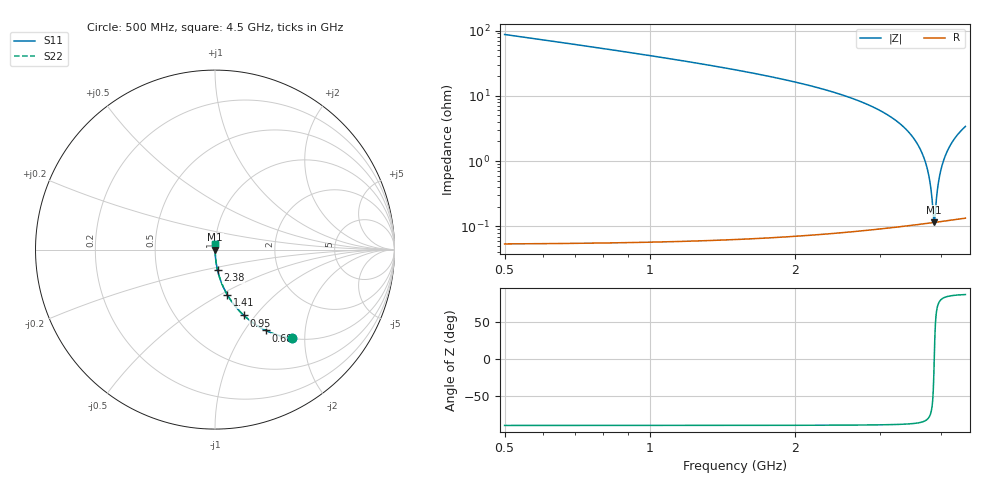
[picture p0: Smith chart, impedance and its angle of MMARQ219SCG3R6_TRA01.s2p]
! MMARQ219SCG3R6_TRA01  S-PARAMETER MODEL  ( General Type )
! Model Generated by TAIYO YUDEN Corporation (http://www.ty-top.com)
! Version 1.0
! TAIYO YUDEN Control No. 180601
! Copyright(c) 2018 TAIYO YUDEN CO.,LTD. All Rights Reserved.
! Product Description (link to TY-COMPAS)
! https://ds.yuden.co.jp/TYCOMPAS/or/detail?pn=MMARQ219SCG3R6BTRA01&u=M
! Products Name : Multilayer Ceramic Capacitors
! Characteristics :
!  Capacitance : 3.6 pF , Rated Voltage : 250V , TCC : CG / C0G
!  Case Size : 2.0 x 1.25 / 0.079 x 0.049 [mm/inch] , Thickness : 0.85 / 0.033 [mm/inch]
!  (Conditions: Temperature = 25 degC , DC Bias Current/Voltage = 0A / 0V)
! External Node Assignments :
!  1  o---| |---o  2
! GND o---------o GND
! Frequency Range : 500MHz  -  4500MHz  [ 401 STEP ]
# MHz S RI R 50
! Freq[MHz].  S11 Real  S11 Imag  S21 Real  S21 Imag  S12 Real  S12 Imag  S22 Real  S22 Imag
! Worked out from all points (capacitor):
!   401 points, 500 MHz to 4.5 GHz, reference 50 ohm
!   read as one part in series: C = 3.6 pF near 520 MHz
!   lowest |Z| = 115 mohm at 3.88 GHz (marker M1)
!   series resonance near 3.879 GHz, so ESL is about 470 pH
!   S11 on the Smith chart (normalised r, x): 500 MHz: 1.00, -1.74; 680 MHz: 1.00, -1.26; 950 MHz: 1.00, -0.87; 1.41 GHz: 1.00, -0.54; 2.38 GHz: 1.00, -0.23; 4.5 GHz: 1.00, +0.07
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500  0.4306 -0.4949  0.5694 0.4949  0.5694 0.4949  0.4306 -0.4949
680  0.2844 -0.4507  0.7156 0.4507  0.7156 0.4507  0.2844 -0.4507
950  0.161 -0.3668  0.839 0.3668  0.839 0.3668  0.161 -0.3668
1170  0.1059 -0.3069  0.8941 0.3069  0.8941 0.3069  0.1059 -0.3069
1410  0.0694 -0.253  0.9306 0.253  0.9306 0.253  0.0694 -0.253
1840  0.0341 -0.1797  0.9659 0.1797  0.9659 0.1797  0.0341 -0.1797
2380  0.014 -0.1141  0.986 0.1141  0.986 0.1141  0.014 -0.1141
2500  0.0113 -0.1021  0.9887 0.1021  0.9887 0.1021  0.0113 -0.1021
3170  0.00309 -0.0461  0.9969 0.0461  0.9969 0.0461  0.00309 -0.0461
3450  0.00174 -0.0267  0.9983 0.0267  0.9983 0.0267  0.00174 -0.0267
3640  0.00129 -0.0144  0.9987 0.0144  0.9987 0.0144  0.00129 -0.0144
3770  0.00116 -0.00646  0.9988 0.00646  0.9988 0.00646  0.00116 -0.00646
3810  0.00115 -0.00406  0.9989 0.00406  0.9989 0.00406  0.00115 -0.00406
3840  0.00114 -0.00228  0.9989 0.00228  0.9989 0.00228  0.00114 -0.00228
3860  0.00114 -0.0011  0.9989 0.0011  0.9989 0.0011  0.00114 -0.0011
3880  0.00115 7.26e-05  0.9989 -7.26e-05  0.9989 -7.26e-05  0.00115 7.26e-05
3890  0.00115 0.000657  0.9988 -0.000657  0.9988 -0.000657  0.00115 0.000657
3940  0.00118 0.00356  0.9988 -0.00356  0.9988 -0.00356  0.00118 0.00356
3970  0.0012 0.00528  0.9988 -0.00528  0.9988 -0.00528  0.0012 0.00528
4070  0.00132 0.0109  0.9987 -0.0109  0.9987 -0.0109  0.00132 0.0109
4250  0.00169 0.0208  0.9983 -0.0208  0.9983 -0.0208  0.00169 0.0208
4500  0.00248 0.0338  0.9975 -0.0338  0.9975 -0.0338  0.00248 0.0338
